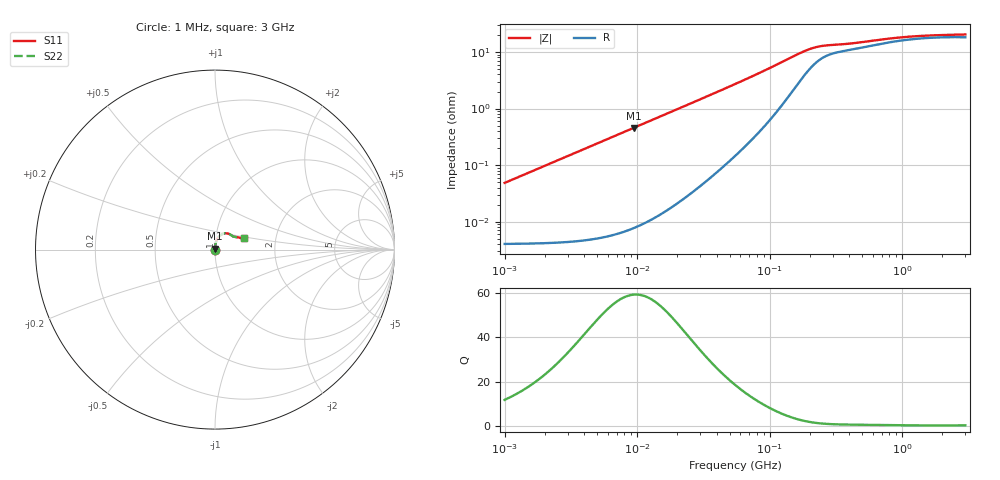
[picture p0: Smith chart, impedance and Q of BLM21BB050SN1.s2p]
! BLM21BB050SN1
# Hz S RI R 50
!Freq.(Hz) S11(Real) S11(Imag) S21(Real) S21(Imag) S12(Real) S12(Imag) S22(Real) S22(Imag)
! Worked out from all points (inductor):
!   401 points, 1 MHz to 3 GHz, reference 50 ohm
!   read as one part in series: L = 7.68 nH near 1.041 MHz
!   highest Q = 59.2 at 9.41 MHz (marker M1), where L = 7.69 nH
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1000000  4.06e-05 0.000483  1 -0.000483  1 -0.000483  4.06e-05 0.000483
1040844  4.07e-05 0.000502  1 -0.000502  1 -0.000502  4.07e-05 0.000502
3823119  4.95e-05 0.00185  1 -0.00185  1 -0.00185  4.95e-05 0.00185
9410094  9.75e-05 0.00454  0.9999 -0.00454  0.9999 -0.00454  9.75e-05 0.00454
1.461624e7  0.000179 0.00706  0.9998 -0.00706  0.9998 -0.00706  0.000179 0.00706
3.065274e7  0.000666 0.0149  0.9993 -0.0149  0.9993 -0.0149  0.000666 0.0149
5.477226e7  0.00217 0.0269  0.9978 -0.0269  0.9978 -0.0269  0.00217 0.0269
8.338914e7  0.00559 0.0418  0.9944 -0.0418  0.9944 -0.0418  0.00559 0.0418
1.244416e8  0.0157 0.064  0.9843 -0.064  0.9843 -0.064  0.0157 0.064
1.520175e8  0.0275 0.0777  0.9725 -0.0777  0.9725 -0.0777  0.0275 0.0777
1.714156e8  0.0383 0.0851  0.9617 -0.0851  0.9617 -0.0851  0.0383 0.0851
1.894586e8  0.0495 0.0894  0.9505 -0.0894  0.9505 -0.0894  0.0495 0.0894
2.094008e8  0.0616 0.0908  0.9384 -0.0908  0.9384 -0.0908  0.0616 0.0908
2.268557e8  0.071 0.0897  0.929 -0.0897  0.929 -0.0897  0.071 0.0897
2.507343e8  0.081 0.0862  0.919 -0.0862  0.919 -0.0862  0.081 0.0862
3.002264e8  0.0928 0.0784  0.9072 -0.0784  0.9072 -0.0784  0.0928 0.0784
4.0536e8  0.1041 0.0719  0.8959 -0.0719  0.8959 -0.0719  0.1041 0.0719
8.005644e8  0.1341 0.0671  0.8659 -0.0671  0.8659 -0.0671  0.1341 0.0671
1.038491e9  0.1441 0.0633  0.8559 -0.0633  0.8559 -0.0633  0.1441 0.0633
1.374365e9  0.1519 0.0597  0.8481 -0.0597  0.8481 -0.0597  0.1519 0.0597
2.050964e9  0.1579 0.0587  0.8421 -0.0587  0.8421 -0.0587  0.1579 0.0587
3e9  0.1591 0.0653  0.8409 -0.0653  0.8409 -0.0653  0.1591 0.0653
